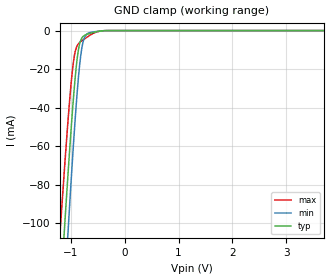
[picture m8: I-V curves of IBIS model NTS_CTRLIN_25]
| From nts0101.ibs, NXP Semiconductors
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|   Model NTS_CTRLIN_25
[Model]   NTS_CTRLIN_25
Model_type   Input
Vinh  =  1.625 | 0.65*Vcc
Vinl  =  0.875 | 0.35*Vcc
C_comp   0.6900pF   0.5232pF   0.9953pF
[Model Spec]
| Note: The input and output voltage ratings may be exceeded if the input and
|   output current ratings are observed (please refer to the data sheet)
|   Subparameter   typ   min   max
Vinh   1.625   1.495   1.755
Vinl   0.875   0.805   0.945
| Overshoot
S_overshoot_high   6.5   6.5   6.5   | Static overshoot
S_overshoot_low   -0.5   -0.5   -0.5
D_overshoot_high   7.2   7.2   7.2   | Dynamic overshoot
D_overshoot_low   -1.0   -1.0   -1.0
D_overshoot_time   3n   3n   3n
|Ambient temperature:   25   85   -40
[Temperature Range]   35   95   -35
[Voltage Range]   2.5   2.3   2.7
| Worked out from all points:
|   GND clamp passes 1 mA (typ) near -0.58 V on its own axis
|Process Range   nominal   slow   fast
[GND_clamp]
|   voltage   I(typ)   I(min)   I(max)
-3V       -1.012A    -1.143A    -900.6mA
-1.2V     -138.9mA   -176.6mA   -104.2mA
-1.12V    -103mA     -136.7mA   -71.92mA
-1.06V    -77.14mA   -107.7mA   -49.04mA
-1.04V    -68.78mA   -98.29mA   -41.85mA
-960mV    -37.6mA    -62.23mA   -17.76mA
-880mV    -13.76mA   -30.86mA   -7.69mA
-820mV    -5.176mA   -13.55mA   -5.806mA
-780mV    -3.231mA   -6.594mA   -4.942mA
-680mV    -1.752mA   -1.375mA   -3.069mA
-340mV    -20.37uA   -28.22uA   -16.89uA
5.5V      0A         0A         0A
